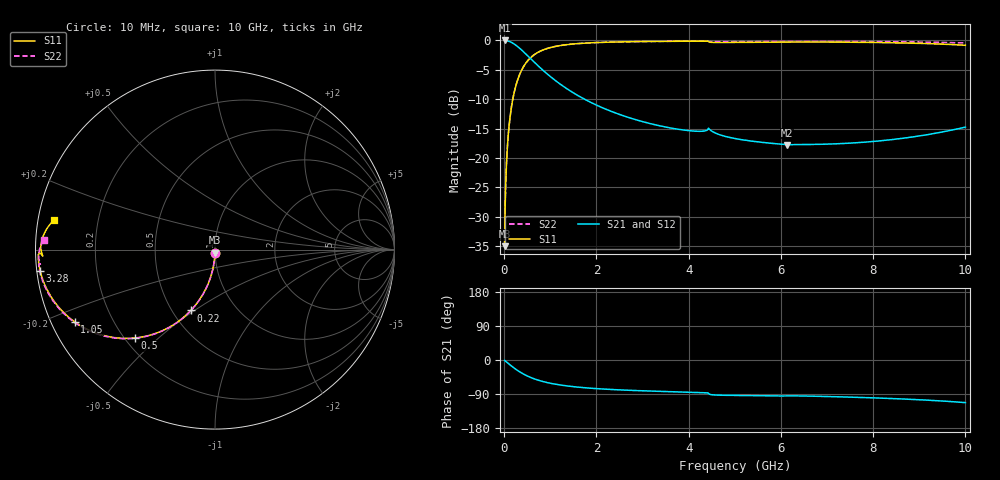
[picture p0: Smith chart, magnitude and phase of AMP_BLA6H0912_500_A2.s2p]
! Created Mon Feb  1 16:20:33 2010
# hz S ma R 50
! 2 Port Network Data from SP1.SP block
! freq  magS11  angS11  magS21  angS21  magS12  angS12  magS22  angS22
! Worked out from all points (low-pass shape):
!   1000 points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, 10 MHz to 10 GHz, reference 50 ohm
!   highest |S21| = 0.00 dB at 10 MHz (marker M1); lowest = -17.8 dB at 6.14 GHz (marker M2)
!   |S21| within 3 dB of the highest: start of sweep to 561.9 MHz
!   lowest |S11| = -35.0 dB at 10 MHz (marker M3), VSWR 1.04, Z = 49.9 - j1.78 ohm
!   |S11| at or under -10 dB: start of sweep to 187.1 MHz
!   |S22| runs from -35.0 to -0.1 dB; largest |S21 - S12| = 0
!   S11 on the Smith chart (normalised r, x): 10 MHz: 1.00, -0.04; 220 MHz: 0.62, -0.48; 500 MHz: 0.24, -0.42; 1.05 GHz: 0.07, -0.24; 3.28 GHz: 0.01, -0.06; 10 GHz: 0.05, +0.09
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1e7  0.01783 -91.0  0.9998 -1.0  0.9998 -1.0  0.01783 -91.0
4e7  0.07116 -94.1  0.9975 -4.1  0.9975 -4.1  0.07116 -94.1
7e7  0.1239 -97.2  0.9923 -7.2  0.9923 -7.2  0.1239 -97.2
1e8  0.1756 -100.2  0.9845 -10.2  0.9845 -10.2  0.1756 -100.2
1.5e8  0.2584 -105.1  0.966 -15.1  0.966 -15.1  0.2584 -105.1
2.2e8  0.365 -111.7  0.931 -21.6  0.931 -21.6  0.365 -111.6
3.4e8  0.5179 -121.6  0.8554 -31.5  0.8554 -31.5  0.5179 -121.4
5e8  0.6643 -132.2  0.7475 -42.1  0.7475 -42.1  0.6643 -132.0
7.5e8  0.7988 -143.9  0.6016 -53.7  0.6016 -53.7  0.7988 -143.5
1.05e9  0.8793 -152.7  0.4762 -62.5  0.4762 -62.5  0.8793 -152.3
1.33e9  0.9183 -158.2  0.3958 -67.9  0.3958 -67.9  0.9183 -157.6
1.68e9  0.9452 -162.9  0.3265 -72.5  0.3265 -72.5  0.9452 -162.2
2.43e9  0.9706 -169.0  0.2405 -78.5  0.2405 -78.5  0.9706 -167.9
3.28e9  0.9814 -173.2  0.1917 -82.4  0.1917 -82.4  0.9814 -171.6
3.34e9  0.9819 -173.4  0.1893 -82.6  0.1893 -82.6  0.9819 -171.8
4.07e9  0.9854 -176.2  0.1701 -85.1  0.1701 -85.1  0.9854 -174.0
4.45e9  0.969 -178.6  0.1758 -90.1  0.1758 -90.1  0.9783 -175.3
5.01e9  0.9625 -178.1  0.1465 -93.5  0.1465 -93.5  0.9787 -175.7
6.14e9  0.97 -179.8  0.1296 -94.6  0.1296 -94.6  0.983 -177.2
6.67e9  0.9707 178.9  0.1306 -95.4  0.1306 -95.4  0.9831 -178.1
8.34e9  0.957 174.9  0.1426 -101.4  0.1426 -101.4  0.9762 179.5
1e10  0.9096 169.5  0.1833 -112.4  0.1833 -112.4  0.9518 176.7
